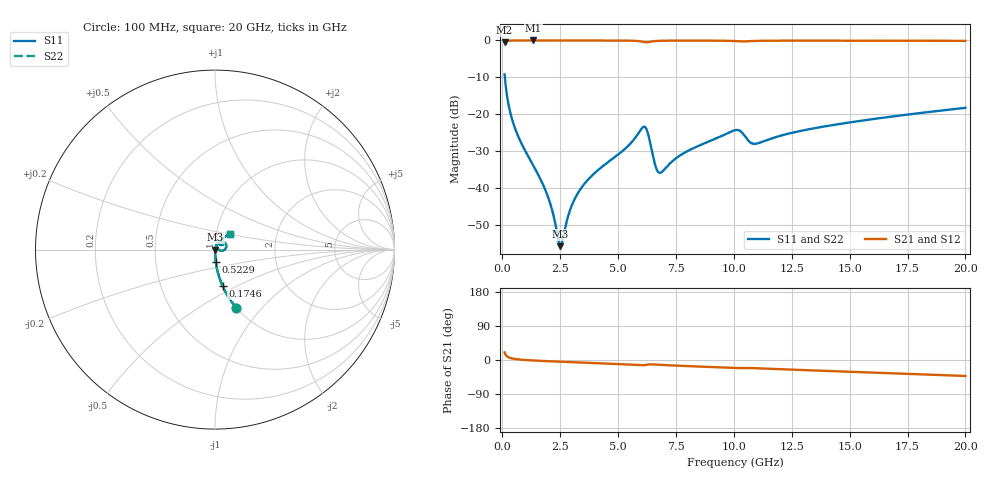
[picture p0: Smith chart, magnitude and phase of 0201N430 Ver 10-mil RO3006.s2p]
# GHz S MA R 50
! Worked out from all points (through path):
!   1601 points, 100 MHz to 20 GHz, reference 50 ohm
!   highest |S21| = -0.01 dB at 1.344 GHz (marker M1); lowest = -0.6 dB at 100 MHz (marker M2)
!   group delay of S21, straight-line fit = 6.09 ps
!   lowest |S11| = -55.9 dB at 2.513 GHz (marker M3), VSWR 1.00, Z = 50.2 - j0.0194 ohm
!   |S11| at or under -10 dB: 110.6 MHz to end of sweep
!   |S22| runs from -55.9 to -9.2 dB; largest |S21 - S12| = 0
!   S11 on the Smith chart (normalised r, x): 100 MHz: 1.00, -0.74; 174.6 MHz: 1.00, -0.42; 522.9 MHz: 1.00, -0.14; 20 GHz: 1.17, +0.20
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0.1  0.3459 -69.9  0.9378 20.1  0.9378 20.1  0.3459 -69.9
0.174625  0.2059 -78.3  0.9781 11.6  0.9781 11.6  0.2059 -78.3
0.323875  0.1115 -83.9  0.9932 5.8  0.9932 5.8  0.1115 -83.9
0.522875  0.0675 -86.5  0.9971 2.9  0.9971 2.9  0.0675 -86.5
1.34375  0.01985 -88.1  0.9987 -1.3  0.9987 -1.3  0.01985 -88.1
1.9905  0.00724 -82.1  0.9985 -3.2  0.9985 -3.2  0.00724 -82.1
2.425813  0.001937 -40.2  0.9984 -4.3  0.9984 -4.3  0.001937 -40.2
2.512875  0.001606 -6.9  0.9983 -4.5  0.9983 -4.5  0.001606 -6.9
2.599937  0.001905 25.9  0.9983 -4.7  0.9983 -4.7  0.001905 25.9
2.973063  0.005449 65.2  0.9981 -5.6  0.9981 -5.6  0.005449 65.2
3.420812  0.01001 71.9  0.9979 -6.7  0.9979 -6.7  0.01001 71.9
5.42325  0.03662 68.7  0.9931 -11.8  0.9931 -11.8  0.03662 68.7
6.107312  0.06717 31.1  0.951 -13.7  0.951 -13.7  0.06717 31.1
6.269  0.05748 3.4  0.9444 -12.1  0.9444 -12.1  0.05748 3.4
6.592375  0.02086 -3.1  0.9792 -12.0  0.9792 -12.0  0.02086 -3.1
6.741625  0.01624 17.5  0.9857 -12.6  0.9857 -12.6  0.01624 17.5
7.9605  0.03094 64.4  0.9942 -16.0  0.9942 -16.0  0.03094 64.4
10.05  0.06039 48.9  0.9776 -21.2  0.9776 -21.2  0.06039 48.9
10.90819  0.03941 45.0  0.9834 -21.5  0.9834 -21.5  0.03941 45.0
13.37081  0.06328 57.9  0.9925 -27.4  0.9925 -27.4  0.06328 57.9
16.69162  0.09127 52.1  0.9904 -34.8  0.9904 -34.8  0.09127 52.1
20  0.1215 45.3  0.9867 -42.1  0.9867 -42.1  0.1215 45.3
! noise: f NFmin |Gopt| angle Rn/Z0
0.1  0.0004447  0.9048  0.2858  0.001025
2.301  0.003712  0.7579  4.147  0.003099
4.515  0.007006  0.7499  8.063  0.005615
6.729  0.01953  0.8584  12.07  0.02918
8.943  0.01414  0.7553  15.91  0.01146
11.14  0.02232  0.8024  19.83  0.02276
13.36  0.01653  0.6998  23.53  0.01034
15.57  0.01748  0.6758  27.24  0.009849
17.79  0.01899  0.6637  30.91  0.01008
20  0.02064  0.656  34.53  0.01047
